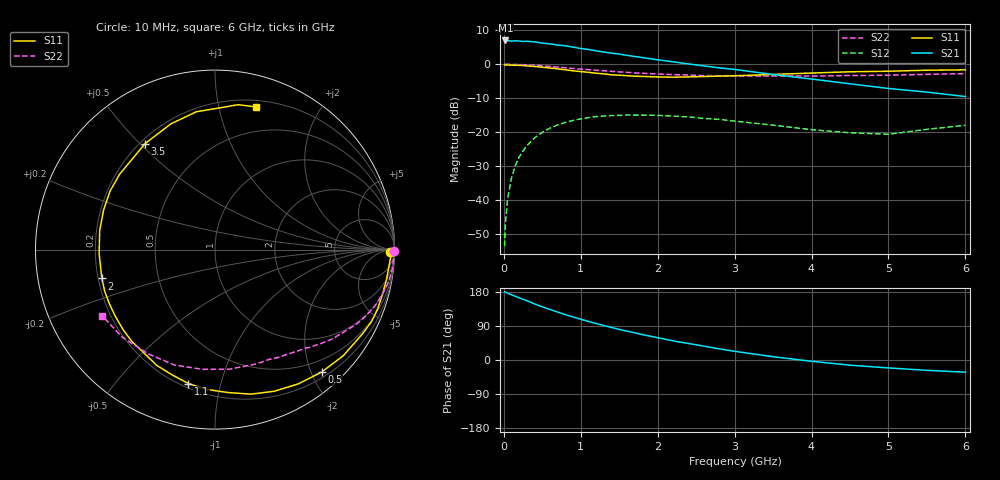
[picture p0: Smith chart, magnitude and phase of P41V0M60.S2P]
! SIEMENS Small Signal Semiconductors
! BFP182
! Si NPN RF Bipolar Junction Transistor in SOT143
! VCE = 1 V  IC = 0.6 mA
! Common Emitter S-Parameters:  March  1996
# GHz  S  MA  R  50
!  f  S11  S21  S12  S22
! GHz  MAG  ANG  MAG  ANG  MAG  ANG  MAG  ANG
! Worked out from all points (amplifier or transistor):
!   36 points, 10 MHz to 6 GHz, reference 50 ohm
!   highest |S21| = 7.0 dB at 20 MHz (marker M1)
!   |S21| within 3 dB of that: start of sweep to 1.184 GHz
!   unconditionally stable (mu >= 1): 2.811 GHz to end of sweep
!   at 250 MHz: K = 0.09, MSG = 16.1 dB, |S12| = -25.5 dB
!   at 1.4 GHz: K = 0.52, MSG = 9.2 dB, |S12| = -15.1 dB
!   at 6 GHz: K = 1.40, MAG = 0.5 dB, |S12| = -18.0 dB
!   S11 on the Smith chart (normalised r, x): 10 MHz: 57, -36; 500 MHz: 0.29, -2.16; 1.1 GHz: 0.22, -0.80; 2 GHz: 0.21, -0.12; 3.5 GHz: 0.22, +0.52; 6 GHz: 0.26, +1.29
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0.01  0.9753 -0.9  2.193 179.7  0.0021 91.6  0.9991 -0.3
0.02  0.9804 -2.2  2.241 179.1  0.0045 88.0  0.9967 -0.8
0.05  0.9745 -5.0  2.237 176.1  0.0107 87.7  0.9977 -1.9
0.1  0.9701 -9.9  2.188 172.1  0.0214 82.8  0.9948 -3.9
0.15  0.9657 -15.2  2.214 168.1  0.0323 79.5  0.9943 -5.9
0.2  0.9646 -20.0  2.198 163.9  0.0432 77.2  0.9905 -7.9
0.3  0.9461 -29.8  2.181 156.5  0.0635 70.4  0.9789 -11.6
0.4  0.9274 -39.6  2.135 147.9  0.0822 64.1  0.9639 -15.3
0.5  0.9047 -49.0  2.049 140.3  0.0996 58.2  0.9479 -18.8
0.6  0.8803 -58.2  1.996 133.3  0.1148 52.5  0.9287 -21.9
0.8  0.83 -76.0  1.872 119.8  0.1393 41.7  0.8885 -28.0
1.1  0.7611 -101.2  1.65 101.5  0.164 28.2  0.8325 -35.4
1.5  0.6903 -132.1  1.414 80.7  0.1769 13.2  0.7712 -43.8
1.8  0.6615 -152.9  1.254 66.9  0.1785 4.9  0.737 -49.0
2  0.6505 -165.7  1.163 58.8  0.177 -0.3  0.7202 -52.6
2.2  0.646 -178.0  1.086 50.5  0.1722 -5.0  0.705 -56.4
2.8  0.6694 150.8  0.885 29.3  0.1544 -15.6  0.679 -67.8
3.5  0.7077 123.4  0.707 8.7  0.127 -21.2  0.6711 -83.3
4.5  0.7753 97.6  0.516 -13.7  0.098 -13.5  0.6817 -109.4
5  0.7892 88.4  0.44 -20.9  0.0933 -1.1  0.6904 -122.9
5.5  0.8174 81.0  0.389 -27.3  0.1103 5.9  0.7107 -136.6
6  0.8271 74.0  0.335 -32.1  0.1262 7.8  0.7286 -149.7
